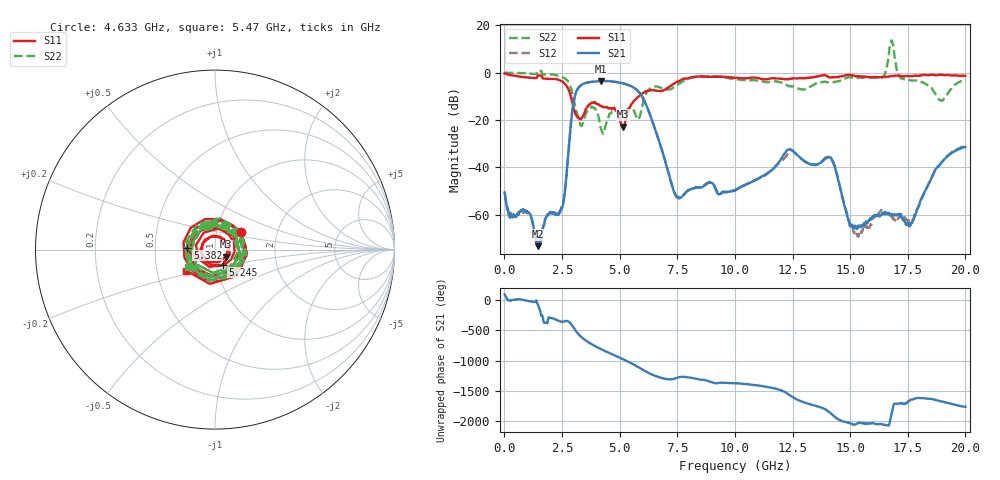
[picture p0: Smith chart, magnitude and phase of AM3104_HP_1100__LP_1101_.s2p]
!Created with skrf (http://scikit-rf.org).
# Hz S RI R 50.0
!freq ReS11 ImS11 ReS21 ImS21 ReS12 ImS12 ReS22 ImS22
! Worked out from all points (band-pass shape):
!   1601 points, 10 MHz to 20 GHz, reference 50 ohm
!   highest |S21| = -3.51 dB at 4.183 GHz (marker M1); lowest = -73.3 dB at 1.459 GHz (marker M2)
!   |S21| within 3 dB of the highest: 3.205 GHz to 5.637 GHz (2.432 GHz wide, 55 % of centre)
!   lowest |S11| = -22.8 dB at 5.132 GHz (marker M3), VSWR 1.16, Z = 56.3 - j4.48 ohm
!   |S11| at or under -10 dB: 2.882 GHz to 5.829 GHz (2.948 GHz wide, 67.7 % of centre)
!   |S22| runs from -25.9 to 13.6 dB; largest |S21 - S12| = 0.07
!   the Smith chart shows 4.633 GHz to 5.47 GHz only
!   S11 on the Smith chart (normalised r, x): 4.633 GHz: 1.30, +0.26; 5.245 GHz: 1.07, -0.18; 5.382 GHz: 0.73, +0.02; 5.47 GHz: 0.71, -0.17
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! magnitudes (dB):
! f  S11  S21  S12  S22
! 10 MHz  -0.4  -50.7  -50.9  0.0
! 1.459 GHz  -1.2  -73.3  -73.3  0.8
! 2.509 GHz  -3.8  -57.1  -56.1  -1.9
! 2.996 GHz  -14.7  -12.9  -12.9  -10.9
! 3.346 GHz  -19.5  -5.2  -5.2  -22.5
! 4.183 GHz  -14.1  -3.5  -3.6  -23.6
! 4.633 GHz  -15.2  -3.7  -3.8  -17.1
! 5.132 GHz  -22.8  -4.5  -4.5  -17.9
! 5.245 GHz  -20.6  -4.8  -4.8  -16.7
! 5.382 GHz  -16.3  -5.3  -5.3  -15.3
! 5.47 GHz  -14.0  -5.6  -5.6  -14.9
! 6.682 GHz  -7.7  -28.0  -28.0  -6.0
! 7.519 GHz  -3.8  -52.9  -52.5  -5.1
! 10.01 GHz  -2.3  -49.9  -49.6  -2.9
! 12.34 GHz  -2.8  -32.6  -33.8  -5.7
! 13.34 GHz  -2.1  -38.9  -38.9  -5.6
! 14.2 GHz  -2.1  -36.6  -36.9  -4.3
! 15.26 GHz  -1.5  -65.7  -68.7  -2.3
! 16.68 GHz  -1.6  -59.5  -59.6  7.2
! 17.6 GHz  -1.5  -64.7  -63.7  -3.2
! 18.95 GHz  -0.9  -38.2  -38.2  -11.8
! 20 GHz  -1.3  -31.5  -31.1  -3.1
